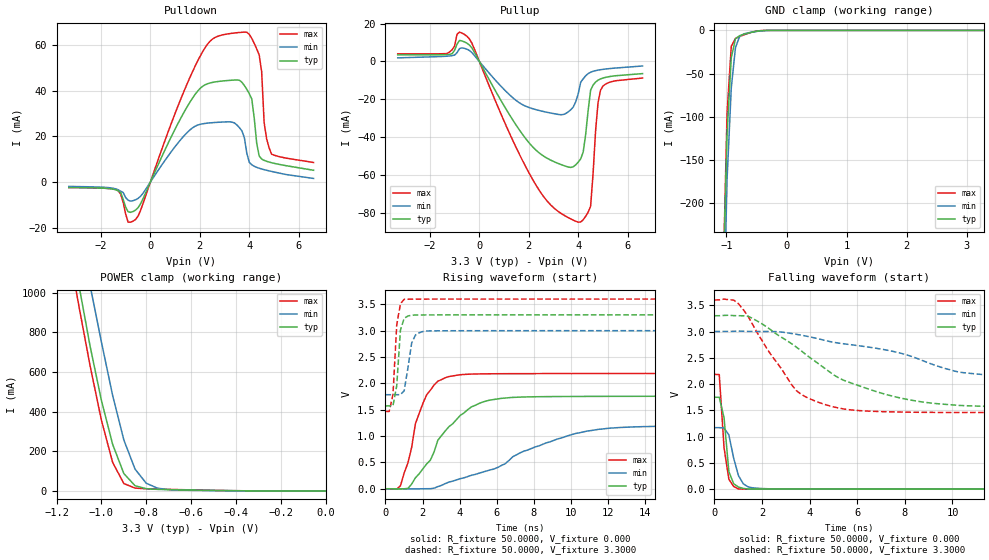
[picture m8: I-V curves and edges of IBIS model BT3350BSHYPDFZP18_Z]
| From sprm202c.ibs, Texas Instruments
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|   Model BT3350BSHYPDFZP18_Z
[Model]   BT3350BSHYPDFZP18_Z
Model_type   I/O
Polarity   Non-Inverting
Enable   Active-Low
Vinl =   1.3000V
Vinh =   1.3000V
Vmeas =   1.6500V
Cref =  15.0000pF
Rref = 100.0000M
Vref =  0.000V
C_comp   1.5700pF   1.6700pF   1.4700pF
[Model Spec]
|   typ   min   max
Vinh   1.37V   1.23V   1.59V
Vinl   1.11V   1.06V   1.23V
[Temperature Range]   25   125   -40
[Voltage Range]   3.30V   3.00V   3.60V
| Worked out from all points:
|   slope of the pulldown table from 0 to 0.495 V, typ, clamps not added: 41.7 ohm
|   slope of the pullup table from 0 to 0.495 V, typ, clamps not added: 41.6 ohm
|   GND clamp passes 1 mA (typ) near -0.50 V on its own axis
|   POWER clamp passes 1 mA (typ) near -0.39 V on its own axis
|   rising waveform, R_fixture 50.0000, V_fixture 0.000: 20-80 % time 2.13ns typ, 4.84ns min, 1.03ns max; typ from 0 V to 1.75 V
|   rising waveform, R_fixture 50.0000, V_fixture 3.3000: 20-80 % time 209ps typ, 323ps min, 219ps max; typ from 1.57 V to 3.3 V
|   falling waveform, R_fixture 50.0000, V_fixture 0.000: 20-80 % time 220ps typ, 389ps min, 257ps max; typ from 1.75 V to 0 V
|   falling waveform, R_fixture 50.0000, V_fixture 3.3000: 20-80 % time 3.87ns typ, 8.72ns min, 1.86ns max; typ from 3.3 V to 1.56 V
[Pulldown]
| voltage   I(typ)   I(min)   I(max)
-3.3V     -2.395mA   -1.898mA   -2.402mA
-1.3V     -3.811mA   -3.398mA   -3.788mA
-900mV    -12.97mA   -7.916mA   -17.55mA
-600mV    -12.26mA   -7.745mA   -16.35mA
2V        40.86mA    25.24mA    54.83mA
3.5V      44.7mA     24.98mA    65.34mA
4.1V      36.36mA    7.585mA    62.87mA
4.4V      11.43mA    6.058mA    55.64mA
4.5V      10.06mA    5.732mA    48.29mA
4.6V      9.513mA    5.439mA    26.03mA
4.9V      8.476mA    4.664mA    12.22mA
6.6V      5.171mA    1.589mA    8.568mA
[Pullup]
| voltage   I(typ)   I(min)   I(max)
-3.3V     3.472mA    1.905mA    4.03mA
-1.3V     3.654mA    2.79mA     4.197mA
-900mV    9.239mA    4.707mA    14.45mA
-500mV    9.64mA     6.478mA    13.31mA
1.9V      -41.21mA   -23.8mA    -56.28mA
3.4V      -54.97mA   -28.03mA   -81.11mA
4V        -53.19mA   -17mA      -84.98mA
4.2V      -47.87mA   -9.179mA   -83.7mA
4.5V      -15.17mA   -5.708mA   -76.52mA
4.7V      -10.89mA   -4.857mA   -36.83mA
4.9V      -9.244mA   -4.36mA    -15.22mA
6.6V      -6.422mA   -2.393mA   -8.759mA
[GND_clamp]
| voltage   I(typ)   I(min)   I(max)
-3.3V     -17.96A    -16.59A    -18.96A
-1.06V    -298.4mA   -373.9mA   -299.7mA
-990mV    -119.9mA   -172.1mA   -95.57mA
-920mV    -31.57mA   -66.47mA   -18.37mA
-850mV    -9.524mA   -19.75mA   -9.271mA
-780mV    -6.103mA   -6.984mA   -7.054mA
-710mV    -4.523mA   -4.047mA   -5.175mA
-640mV    -3.174mA   -2.833mA   -3.436mA
-500mV    -1.042mA   -1.202mA   -810.1uA
-360mV    -137uA     -246.4uA   -55.55uA
3.28V     93.14nA    68.38uA    379.5nA
[POWER_clamp]
| voltage   I(typ)   I(min)   I(max)
-3.3V     16.8A      15.72A     17.64A
-1.15V    1.371A     1.626A     1.251A
-1.1V     1.036A     1.326A     930.2mA
-1.05V    727.4mA    1.034A     628.7mA
-1V       456.7mA    751.2mA    357mA
-950mV    235.1mA    481.7mA    143.9mA
-900mV    87.54mA    256.7mA    37.14mA
-850mV    26.08mA    109.7mA    14.26mA
-800mV    11.15mA    38.59mA    10.64mA
-750mV    7.763mA    13.84mA    9.099mA
-650mV    5.352mA    4.02mA     6.499mA
0V        96.18nA    60.17nA    426.3nA
[Ramp]
| variable   typ   min   max
dV/dt_r   1.0532/2.1340n   0.7119/4.8566n   1.3130/1.0475n
dV/dt_f   1.0459/3.8275n   0.6029/6.1142n   1.2837/1.8424n
R_load = 50.0000
[Rising Waveform]
R_fixture = 50.0000
V_fixture = 0.000
V_fixture_min = 0.000
V_fixture_max = 0.000
| time   V(typ)   V(min)   V(max)
0s        8.394uV    2.658uV    13.65uV
808.1ps   -4.953mV   -72.6uV    55.18mV
1.414ns   88.93mV    -3.431mV   786.6mV
1.616ns   208.2mV    -2.086mV   1.235V
2.222ns   469.8mV    557uV      1.782V
3.434ns   1.181V     127.3mV    2.13V
5.657ns   1.684V     358.4mV    2.182V
7.475ns   1.742V     714mV      2.185V
10.91ns   1.753V     1.096V     2.187V
20ns      1.755V     1.186V     2.188V
[Rising Waveform]
R_fixture = 50.0000
V_fixture = 3.3000
V_fixture_min = 3.0000
V_fixture_max = 3.6000
| time   V(typ)   V(min)   V(max)
0s        1.573V     1.784V     1.468V
202ps     1.573V     1.785V     1.468V
404ps     1.575V     1.785V     1.786V
606.1ps   1.952V     1.785V     3.105V
808.1ps   3.012V     1.785V     3.511V
1.01ns    3.236V     1.86V      3.595V
1.414ns   3.295V     2.765V     3.598V
1.616ns   3.297V     2.916V     3.599V
2.02ns    3.298V     2.984V     3.599V
20ns      3.3V       3V         3.6V
[Falling Waveform]
R_fixture = 50.0000
V_fixture = 0.000
V_fixture_min = 0.000
V_fixture_max = 0.000
| time   V(typ)   V(min)   V(max)
0s        1.748V     1.171V     2.183V
202ps     1.749V     1.171V     2.181V
404ps     1.357V     1.164V     785.7mV
606.1ps   332.8mV    1.031V     189.1mV
808.1ps   102.1mV    589mV      50.71mV
1.01ns    39.9mV     255.3mV    4.433mV
1.212ns   13.84mV    101.9mV    928.4uV
1.414ns   3.324mV    43.46mV    750.7uV
2.424ns   445.1uV    5.042mV    184.8uV
20ns      -1.655uV   12.43uV    -1.647uV
[Falling Waveform]
R_fixture = 50.0000
V_fixture = 3.3000
V_fixture_min = 3.0000
V_fixture_max = 3.6000
| time   V(typ)   V(min)   V(max)
0s        3.3V       3V         3.6V
808.1ps   3.302V     3.003V     3.598V
1.01ns    3.3V       3.008V     3.528V
1.616ns   3.246V     3.001V     3.124V
3.434ns   2.705V     2.947V     1.879V
5.051ns   2.163V     2.791V     1.56V
7.273ns   1.794V     2.643V     1.473V
9.495ns   1.621V     2.323V     1.46V
10.51ns   1.589V     2.215V     1.46V
20ns      1.557V     1.789V     1.461V
